// ------------------------------------------------------------------
// File           : C:\Documents and Settings\XP\Desktop\FCA\TO.awl
//
// Source File    : C:\Documents and Settings\XP\Desktop\FCA\TO.var
// Generation Date: 04/09/2017  Time: 13:44:46
// ------------------------------------------------------------------

DATA_BLOCK DB  120
VERSION : 0.0


STRUCT

 T1_TO_cuttEdgeParam29_2:
   STRUCT
   SYNTAX_ID : BYTE  := B#16#82;
   bereich_u_einheit : BYTE := B#16#81;
   spalte : WORD := W#16#2;
   zeile : WORD := W#16#1D;
   bausteintyp : BYTE := B#16#14;
   ZEILENANZAHL : BYTE := B#16#1;
   typ : BYTE := B#16#F;
   laenge : BYTE := B#16#8;
   END_STRUCT ;

 END_STRUCT ;

BEGIN
END_DATA_BLOCK
